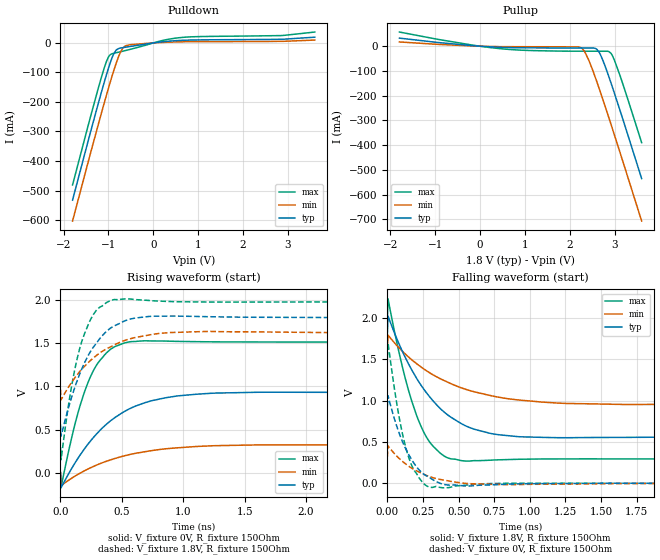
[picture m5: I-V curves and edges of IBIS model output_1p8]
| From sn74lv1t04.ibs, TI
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|   output_1p8 Model
[Model]   output_1p8
Model_type   Output
Polarity   Inverting
Vmeas = 0.9
Vref = 0
Cref = 30pF
Rref = 500
|   typ   min   max
|   (nom PVT)   (fast PVT)   (slow PVT)
C_comp   2.219e-12   2.168e-12   2.314e-12
| Where nom  PVT is Nominal Process, 1.8V, 40C
|   Fast PVT is Strong Process,  1.98V, -40C
|   Slow PVT is Weak Process,   1.62V, 140C
[Voltage Range]   1.8   1.62   1.98
|Junction Temperature
[Temperature Range]   40   140   -40
[Pullup Reference]   1.8   1.62   1.98
[Pulldown Reference]   0   0   0
[Power Clamp Reference]   1.8   1.62   1.98
[GND Clamp Reference]   0   0   0
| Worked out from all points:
|   slope of the pulldown table from 0 to 0.27 V, typ, clamps not added: 54.9 ohm
|   slope of the pullup table from 0 to 0.27 V, typ, clamps not added: 91.8 ohm
|   falling waveform, V_fixture 1.8V, R_fixture 150Ohm: 20-80 % time 321ps typ, 459ps min, 178ps max; typ from 1.8 V to 0.561 V
|   rising waveform, V_fixture 0V, R_fixture 150Ohm: 20-80 % time 411ps typ, 475ps min, 205ps max; typ from 0 V to 0.926 V
|   rising waveform, V_fixture 1.8V, R_fixture 150Ohm: 20-80 % time 242ps typ, 334ps min, 155ps max; typ from 0.561 V to 1.8 V
|   falling waveform, V_fixture 0V, R_fixture 150Ohm: 20-80 % time 155ps typ, 214ps min, 108ps max; typ from 0.926 V to 0 V
[Pulldown]
|   Voltage   I(typ)   I(min)   I(max)
-1.8V     -532.5mA   -603.3mA   -481.1mA
-1.232V   -207.8mA   -279.2mA   -156.2mA
-1.044V   -107.4mA   -176.5mA   -62.59mA
-966.4mV  -70.11mA   -136mA     -40.77mA
-887.4mV  -38.57mA   -96.5mA    -35.33mA
-831.6mV  -24.73mA   -70.45mA   -33.33mA
-722.7mV  -17.01mA   -28.54mA   -29.49mA
-651.4mV  -15.18mA   -13.03mA   -26.9mA
-518.6mV  -12.01mA   -5.989mA   -21.92mA
623.5mV   8.739mA    3.861mA    18.46mA
2.841V    12.34mA    5.369mA    24.93mA
3.6V      19.53mA    9.748mA    37mA
[Pullup]
|   Voltage   I(typ)   I(min)   I(max)
-1.8V     32.8mA     17.27mA    57.44mA
360mV     -3.713mA   -1.426mA   -8.193mA
2.19V     -7.081mA   -2.688mA   -20.07mA
2.278V    -7.092mA   -10.14mA   -20.11mA
2.428V    -7.11mA    -59.42mA   -20.18mA
2.601V    -12.18mA   -143.7mA   -20.25mA
2.709V    -45.34mA   -201.2mA   -20.3mA
2.844V    -110.2mA   -275.4mA   -20.36mA
2.918V    -149.5mA   -316.9mA   -29.07mA
2.994V    -190.4mA   -359.3mA   -56.64mA
3.112V    -256.6mA   -426.8mA   -115.9mA
3.6V      -535.5mA   -707.3mA   -390.1mA
[Ramp]
R_load = 150
|   typ   min   max
dV/dt_r   0.555531/4.11224e-10   0.189893/4.76039e-10   0.909385/2.04682e-10
dV/dt_f   0.743446/3.20868e-10   0.393173/4.59916e-10   1.01154/1.78013e-10
[Falling Waveform]
V_fixture = 1.8V
V_fixture_min = 1.62V
V_fixture_max = 1.98V
R_fixture = 150Ohm
|   Time   V(typ)   V(min)   V(max)
0s        1.8V       1.62V      1.98V
5ps       2.019V     1.788V     2.227V
125ps     1.523V     1.563V     1.274V
235ps     1.188V     1.407V     694.1mV
320ps     997.3mV    1.311V     450.5mV
445ps     800.2mV    1.204V     296.8mV
620ps     648.7mV    1.101V     273.9mV
935ps     561.8mV    1.004V     291mV
1.665ns   554.6mV    952.1mV    294.7mV
4.615ns   561.2mV    965.1mV    294.1mV
[Rising Waveform]
V_fixture = 0V
V_fixture_min = 0V
V_fixture_max = 0V
R_fixture = 150Ohm
|   Time   V(typ)   V(min)   V(max)
0s        379.3pV    7.523nV    458.2pV
5ps       -176.4mV   -150.5mV   -171mV
80ps      20.61mV    -75.23mV   334.8mV
145ps     171.6mV    -18.07mV   704.7mV
270ps     409.9mV    72.81mV    1.187V
405ps     597.7mV    146.2mV    1.427V
550ps     731.7mV    205.3mV    1.514V
860ps     868.9mV    277.1mV    1.526V
1.275ns   923mV      313.1mV    1.517V
5.645ns   925.6mV    316.3mV    1.516V
[Rising Waveform]
V_fixture = 1.8V
V_fixture_min = 1.62V
V_fixture_max = 1.98V
R_fixture = 150Ohm
|   Time   V(typ)   V(min)   V(max)
0s        560.9mV    964.7mV    294.1mV
5ps       423.2mV    843.8mV    149mV
90ps      870.2mV    1.045V     995.7mV
135ps     1.062V     1.133V     1.315V
175ps     1.206V     1.201V     1.527V
290ps     1.496V     1.356V     1.878V
410ps     1.678V     1.46V      1.997V
605ps     1.792V     1.566V     2.008V
900ps     1.816V     1.626V     1.984V
3.285ns   1.8V       1.619V     1.98V
[Falling Waveform]
V_fixture = 0V
V_fixture_min = 0V
V_fixture_max = 0V
R_fixture = 150Ohm
|   Time   V(typ)   V(min)   V(max)
0s        925.9mV    316.5mV    1.516V
5ps       1.058V     452.8mV    1.696V
75ps      645.4mV    314mV      875.2mV
110ps     488.8mV    259.8mV    570mV
145ps     365mV      213.1mV    339.8mV
190ps     234.9mV    164.2mV    153mV
290ps     77.9mV     85.42mV    -42.53mV
400ps     -13.9mV    38.93mV    -54.36mV
560ps     -31.68mV   -1.872mV   -20.65mV
2.965ns   -72.85uV   617uV      -33.77uV
